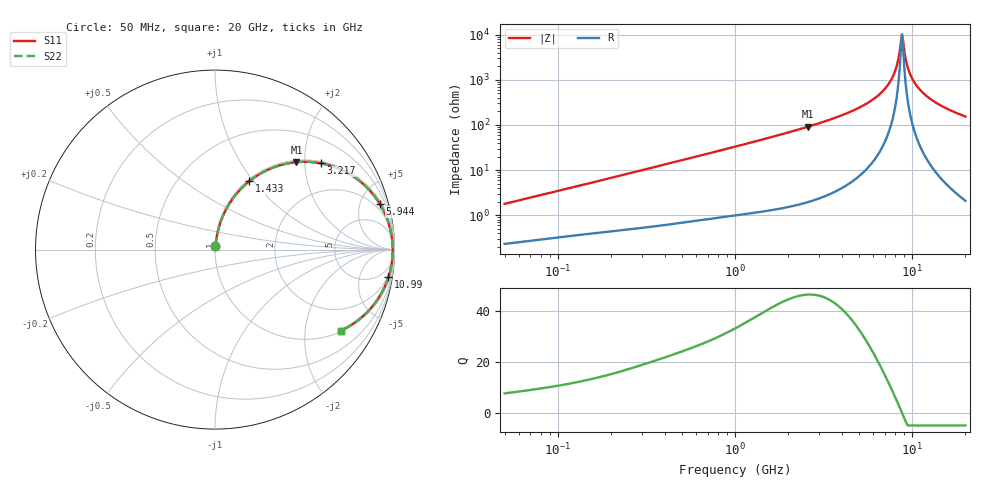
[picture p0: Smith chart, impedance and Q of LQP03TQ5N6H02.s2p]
!Murata Part Number: LQP03TQ5N6H02
!These Parameters are Measured in Series Mode Connection
!  o--[Z]--o
!Port1  Port2
!  o-------o
!Freq. Start=50[MHz] Stop=20[GHz], 401[Steps]
# Hz S RI R 50
!Freq.(Hz) S11(Real) S11(Imag) S21(Real) S21(Imag) S12(Real) S12(Imag) S22(Real) S22(Imag)
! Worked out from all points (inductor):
!   401 points, 50 MHz to 20 GHz, reference 50 ohm
!   read as one part in series: L = 5.61 nH near 51.52 MHz
!   highest Q = 46.5 at 2.569 GHz (marker M1), where L = 5.63 nH
!   self-resonance near 8.645 GHz
!   S11 on the Smith chart (normalised r, x): 50 MHz: 1.00, +0.04; 1.433 GHz: 1.02, +0.96; 3.217 GHz: 1.05, +2.40; 5.944 GHz: 1.29, +7.09; 10.99 GHz: 2, -12; 20 GHz: 1.04, -3.08
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5e7  0.00265 0.0177  0.9974 -0.0177  0.9974 -0.0177  0.00265 0.0177
1.364002e8  0.00587 0.0461  0.9941 -0.0461  0.9941 -0.0461  0.00587 0.0461
3.721004e8  0.0207 0.1205  0.9793 -0.1205  0.9793 -0.1205  0.0207 0.1205
1e9  0.1056 0.2927  0.8944 -0.2927  0.8944 -0.2927  0.1056 0.2927
1.432596e9  0.1922 0.3815  0.8078 -0.3815  0.8078 -0.3815  0.1922 0.3815
2.569357e9  0.4538 0.4872  0.5462 -0.4872  0.5462 -0.4872  0.4538 0.4872
2.728004e9  0.4887 0.4892  0.5113 -0.4892  0.5113 -0.4892  0.4887 0.4892
3.216634e9  0.589 0.4811  0.411 -0.4811  0.411 -0.4811  0.589 0.4811
4.539627e9  0.7941 0.391  0.2059 -0.391  0.2059 -0.391  0.7941 0.391
5.944466e9  0.9175 0.2554  0.0825 -0.2554  0.0825 -0.2554  0.9175 0.2554
6.802353e9  0.9584 0.172  0.0416 -0.172  0.0416 -0.172  0.9584 0.172
7.442007e9  0.9766 0.1127  0.0234 -0.1127  0.0234 -0.1127  0.9766 0.1127
8.020766e9  0.986 0.0619  0.014 -0.0619  0.014 -0.0619  0.986 0.0619
8.264682e9  0.9883 0.0413  0.0117 -0.0413  0.0117 -0.0413  0.9883 0.0413
8.516016e9  0.9896 0.0206  0.0104 -0.0206  0.0104 -0.0206  0.9896 0.0206
8.774992e9  0.9901 -9.84e-05  0.00986 9.84e-05  0.00986 9.84e-05  0.9901 -9.84e-05
8.907419e9  0.9901 -0.0105  0.00993 0.0105  0.00993 0.0105  0.9901 -0.0105
9.316812e9  0.9885 -0.0415  0.0115 0.0415  0.0115 0.0415  0.9885 -0.0415
9.745021e9  0.9851 -0.0724  0.0149 0.0724  0.0149 0.0724  0.9851 -0.0724
1.098561e10  0.9664 -0.1531  0.0336 0.1531  0.0336 0.1531  0.9664 -0.1531
1.396067e10  0.8901 -0.2996  0.1099 0.2996  0.1099 0.2996  0.8901 -0.2996
2e10  0.7008 -0.4511  0.2992 0.4511  0.2992 0.4511  0.7008 -0.4511
